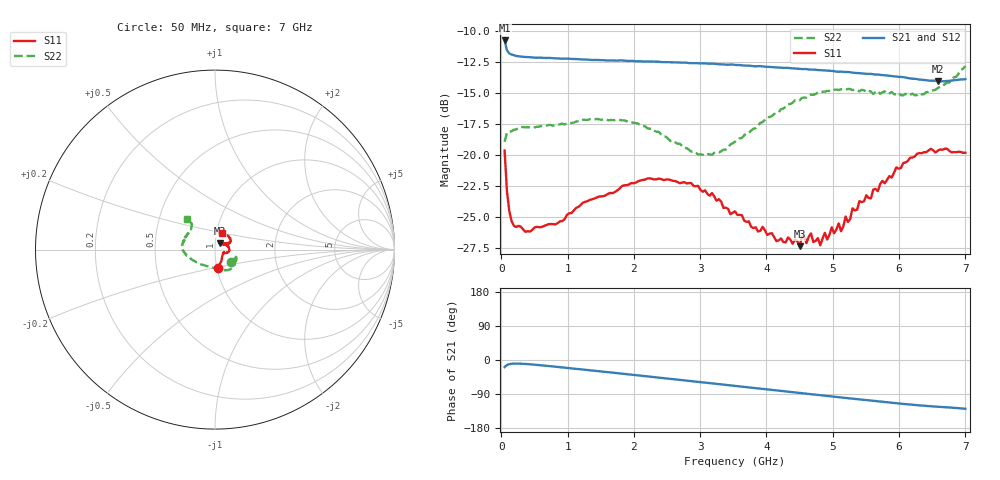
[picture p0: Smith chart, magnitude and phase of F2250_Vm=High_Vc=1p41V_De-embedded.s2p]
! Integrated Device Technology
! Corporate Headquarters
! 6024 Silver Creek Valley Road
! San Jose, CA 95138  USA
! Phone:  1-408-284-8200
! Toll Free:  1-800-223-1366
! Webpage:  http://www.idt.com/
! Timing and RF Division
! 515 Groton Road, Suite 102
! Westford, MA 01886-6024
! Device:  F2250
! Description: Voltage Variable RF Attenuator
! Frequency:  50.0 -  6000.00 MHz
! Package:  3x3 mm Thin QFN Plastic Package: 16 pin
! Ports:  2 RF, 3 DC
!  Pin  1  = GND
!  Pin  2  = NC
!  Pin  3  = RF1  = Port 1
!  Pin  4  = NC
!  Pin  5  = GND
!  Pin  6  = GND
!  Pin  7  = GND
!  Pin  8  = GND
!  Pin  9  = NC
!  Pin 10  = RF2  = Port 2
!  Pin 11  = NC
!  Pin 12  = GND
!  Pin 13  = GND
!  Pin 14  = VCNTRL
!  Pin 15  = VDD
!  Pin 16  = VMODE
! Vcntrl:  1.410 Volts
! Vmode:  +3.300 Volts
! Vdd:  +3.30  Volts
! Current:  1.331 mA
! Data:  The device was measured on a the F2250 evaluation board which has
!  individual transmission lines to the RF pins.  Data was collected
!  using a calibrated network analyzer.  The evaluation board was
!  de-embedded using a TRL calibration technique.
!  The reference plane is the edge of the package pin.
! Misc:  SN 10
!  Action Tracker AT0258
! Date Measured:  2014-11-26
! Date:  2015-10-15  MJV
! Note:
!  Integrated Device Technology supplies this data as a sample of measured
!  data at the package pin for this product.  Your particular data for this
!  product may vary.
!  Data was taken at 25 degrees C.
!  Integrated Device Technology reserves the right to change this data at anytime.
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# GHz S dB R 50
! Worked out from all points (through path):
!   201 points, 50 MHz to 7 GHz, reference 50 ohm
!   highest |S21| = -10.73 dB at 50 MHz (marker M1); lowest = -14.1 dB at 6.583 GHz (marker M2)
!   group delay of S21, straight-line fit = 51 ps
!   lowest |S11| = -27.4 dB at 4.498 GHz (marker M3), VSWR 1.09, Z = 52.5 + j3.59 ohm
!   |S11| at or under -10 dB: start of sweep to end of sweep
!   |S22| runs from -20.0 to -12.8 dB; largest |S21 - S12| = 0.0012
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0.05  -19.63 -81.3  -10.73 -18.5  -10.71 -18.5  -18.93 -39.3
0.08475  -22.86 -60.3  -11.52 -13.3  -11.52 -13.3  -18.18 -21.7
0.1195  -24.49 -49.5  -11.78 -11.0  -11.78 -11.0  -18.11 -16.4
0.189  -25.70 -34.8  -11.93 -9.5  -11.94 -9.5  -17.96 -14.4
0.8145  -25.61 -16.5  -12.18 -17.7  -12.19 -17.7  -17.60 -29.7
1.2315  -23.85 -17.6  -12.27 -25.2  -12.27 -25.2  -17.14 -41.3
2.37825  -21.90 -0.4  -12.45 -46.4  -12.47 -46.5  -18.12 -67.5
3.07325  -22.84 17.5  -12.58 -59.8  -12.59 -59.8  -20.03 -103.2
3.525  -24.55 32.8  -12.71 -68.4  -12.72 -68.5  -18.92 -133.4
3.8725  -26.18 45.5  -12.81 -75.0  -12.81 -75.1  -17.62 -151.7
4.498  -27.36 52.7  -13.02 -87.0  -13.03 -87.0  -15.58 -172.4
4.67175  -26.33 53.9  -13.09 -90.3  -13.08 -90.4  -15.11 -176.1
4.7065  -27.03 54.3  -13.09 -91.0  -13.09 -91.0  -15.14 -176.8
4.81075  -27.29 49.5  -13.13 -92.9  -13.13 -92.9  -14.89 -178.7
4.88025  -26.28 47.4  -13.15 -94.3  -13.16 -94.3  -14.87 179.2
5.08875  -25.52 41.2  -13.26 -98.2  -13.23 -98.3  -14.74 174.7
5.1235  -26.15 40.9  -13.25 -98.9  -13.22 -99.0  -14.67 173.7
5.29725  -24.30 31.9  -13.33 -102.1  -13.33 -102.1  -14.75 170.2
5.85325  -21.69 25.0  -13.59 -112.2  -13.59 -112.4  -15.01 155.2
6.27025  -19.89 29.6  -13.86 -119.2  -13.87 -119.2  -15.15 142.2
6.583  -19.65 39.6  -14.05 -123.3  -14.03 -123.5  -14.58 133.7
7  -19.81 68.5  -13.86 -128.7  -13.87 -128.8  -12.80 132.6
